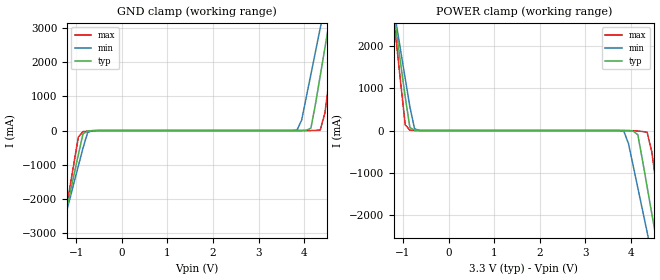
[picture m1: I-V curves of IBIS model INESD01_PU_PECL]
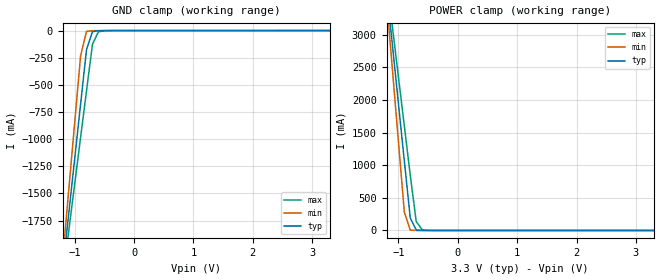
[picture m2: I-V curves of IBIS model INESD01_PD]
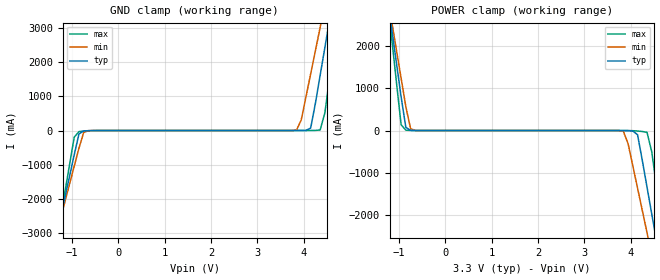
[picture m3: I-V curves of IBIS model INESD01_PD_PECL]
|   This file is an IBIS representation of the   |
|   Integrated Device Technology , Inc.   |
|   ICS87951I   |
|   LOW SKEW, 1-TO-9 DIFFERENTIAL-TO-LVCMOS/LVTTL ZERO DELAY BUFFER   |
[IBIS Ver]   4.1
[File name]   87951i_3v3.ibs
[File Rev]   1.0
[Date]   22 Jun 2009 | Last modified
[Source]   Originated at Integrated Device Technology, Inc.
[Disclaimer]
IDT hereby grants the user of this IBIS model a non-exclusive,
nontransferable license to use this IBIS model under the following terms.
Before using this IBIS model, the user should read this license.
If the user does not accept these terms,  the IBIS model should be
returned to IDT within 30 days.
   The user is granted this license only to use the IBIS model and
is not granted rights to sell, load, rent, lease or license the IBIS
model in whole or in part, or in modified form to anyone other than
user. User may modify the IBIS model to suit its specific
applications but rights to derivative works and such modifications
shall belong to IDT.
   This IBIS model is provided on an "AS IS" basis and IDT makes
absolutely no warranty with respect to the information contained
herein. IDT DISCLAIMS AND CUSTOMER WAIVES ALL WARRANTIES, EXPRESS
OR IMPLIED, INCLUDING WARRANTIES OF MERCHANTABILITY OR FITNESS FOR
A PARTICULAR PURPOSE. The entire risk as to quality and performance
is with the Customer. ACCORDINGLY, IN NO EVENT SHALL THE COMPANY BE
LIABLE FOR ANY DAMAGES, WHETHER IN CONTRACT OR TORT,INCLUDING ANY
LOST PROFITS OR OTHER INCIDENTAL, CONSEQUENTIAL, EXEMPLARY, OR
PUNITIVE DAMAGES ARISING OUT OF THE USE OR APPLICATION OF THE IBIS
model provided in this package. Further, IDT reserves the right to
make changes without notice to any product herein to improve
reliability, function, or design. IDT does not convey any license
under patent rights or any other intellectual property rights,
including those of third parties.
   IDT is not obligated to provide maintenance or support
for the licensed IBIS model.
[Copyright]   Copyright 2003 by Integrated Device Technology , Inc.
[Component]   ICS87951i
[Manufacturer] Integrated Device Technology, Inc.
[Package]
|LQFP32
|lead + wire   typ   min   max
R_pkg   220.4m   212.5m   238m
L_pkg   1.841nH   1.708nH   1.974n
C_pkg   0.316pF   0.2907pF   0.33pF
[Pin] signal_name   model_name   R_pin   L_pin   C_pin
1   VDDA   POWER   238m   1.974n   0.330p
2   EXT_FB   INESD01_PU_PECL   225m   1.841n   0.311p
3   DIV_SELA   INESD01_PD   218m   1.7745n   0.301p
4   DIV_SELB   INESD01_PD   213m   1.708n   0.291p
5   DIV_SELC   INESD01_PD   213m   1.708n   0.291p
6   DIV_SELD   INESD01_PD   218m   1.7745n   0.301p
7   GND   GND   225m   1.841n   0.311p
8   CLK1   INESD01_PU_PECL   238m   1.974n   0.330p
9   nCLK1   INESD01_PD_PECL   238m   1.974n   0.330p
10   MR/nOE   INESD01_PD   225m   1.841n   0.311p
11   VDDO   POWER   218m   1.7745n   0.301p
12   QD4   COUT05   213m   1.708n   0.291p
13   GND   GND   213m   1.708n   0.291p
14   QD3   COUT05   218m   1.7745n   0.301p
15   VDDO   POWER   225m   1.841n   0.311p
16   QD2   COUT05   238m   1.974n   0.330p
17   GND   GND   238m   1.974n   0.330p
18   QD1   COUT05   225m   1.841n   0.311p
19   VDDO   POWER   218m   1.7745n   0.301p
20   QD0   COUT05   213m   1.708n   0.291p
21   GND   GND   213m   1.708n   0.291p
22   QC1   COUT05   218m   1.7745n   0.301p
23   VDDO   POWER   225m   1.841n   0.311p
24   QC0   COUT05   238m   1.974n   0.330p
25   GND   GND   238m   1.974n   0.330p
26   QB   COUT05   225m   1.841n   0.311p
27   VDDO   POWER   218m   1.7745n   0.301p
28   QA   COUT05   213m   1.708n   0.291p
29   GND   GND   213m   1.708n   0.291p
30   CLK0   INESD01_PD_PECL   218m   1.7745n   0.301p
31   PLL_SEL   INESD01_PD   225m   1.841n   0.311p
32   CLK_SEL   INESD01_PD   238m   1.974n   0.330p
[Diff Pin]   inv_pin   vdiff   tdelay_typ   tdelay_min   tdelay_max
8   9   0.30   0   0   0
| Models and submodels in the file (4): INESD01_PU_PECL (Input), INESD01_PD (Input), INESD01_PD_PECL (Input), COUT05 (Output)
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[Model]   INESD01_PU_PECL
Model_type  Input
Polarity   Non-Inverting
Vinl = 0.8V
Vinh = 2.0V
|   typ   min   max
C_comp   2pF   1.5pF   2.5pF
|   typ   min   max
[Voltage range]  3.3V   3.15V   3.45V
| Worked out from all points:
|   GND clamp passes 1 mA (typ) near -0.55 V on its own axis
|   POWER clamp passes 1 mA (typ) near -0.67 V on its own axis
[GND_clamp]
|Voltage   I(typ)   I(min)   I(max)
-3.3V     -15.3A     -13.19A    -18.82A
-1.361V   -3.24A     -3.145A    -3.432A
-1.259V   -2.606A    -2.617A    -2.622A
-952.6mV  -705.4mA   -1.038A    -192.5mA
-850.5mV  -99.96mA   -513.6mA   -31.29mA
-646.4mV  -3.852mA   -3.611mA   -8.361mA
3.844V    64.83uA    13.07mA    7.183uA
4.151V    73.26mA    1.652A     800.8uA
4.355V    1.607A     3.003A     15.37mA
4.559V    3.233A     4.356A     1.553A
4.763V    4.861A     5.711A     3.635A
6.6V      19.56A     17.94A     22.42A
[POWER_clamp]
|Voltage   I(typ)   I(min)   I(max)
-3.3V     19.56A     16.84A     24.11A
-1.259V   3.233A     3.262A     3.235A
-1.157V   2.419A     2.586A     2.194A
-952.6mV  795.8mA    1.236A     137.7mA
-850.5mV  73.26mA    563.1mA    8.081mA
-646.4mV  471.5uA    1.942mA    367.2uA
3.844V    -890.5uA   -18.21mA   -111uA
4.151V    -99.96mA   -1.362A    -11.88mA
4.355V    -1.338A    -2.415A    -41.77mA
4.559V    -2.606A    -3.47A     -1.313A
4.763V    -3.875A    -4.526A    -2.933A
6.6V      -15.3A     -14.05A    -17.51A
[Model]   INESD01_PD
Model_type   Input
Polarity   Non-Inverting
Vinl = 0.80V
Vinh = 2.0V
|   typ   min   max
C_comp   2pF   1.5pF   2.5pF
|   typ   min   max
[Voltage range]  3.3V   3.15V   3.45V
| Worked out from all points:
|   GND clamp passes 1 mA (typ) near -0.55 V on its own axis
|   POWER clamp passes 1 mA (typ) near -0.60 V on its own axis
[GND_clamp]
|Voltage I(typ)   I(min)   I(max)
-3.3V     -12.83A    -15.14A    -11.37A
-1.2V     -2.195A    -2.092A    -2.281A
-1.1V     -1.689A    -1.472A    -1.849A
-900mV    -678.5mA   -232.6mA   -984.8mA
-800mV    -173.9mA   -7.175mA   -553.2mA
-700mV    -9.696mA   -1.052mA   -126mA
-600mV    -1.629mA   -178uA     -11.07mA
-300mV    -10.53uA   -5.678uA   -86.08uA
3.3V      71.13uA    62.11uA    77.58uA
[POWER_clamp]
|Voltage   I(typ)   I(min)   I(max)
-3.3V     22.38A     26.45A     19.82A
-1.2V     3.723A     3.545A     3.874A
-1.1V     2.836A     2.457A     3.116A
-1V       1.949A     1.369A     2.358A
-900mV    1.063A     281.1mA    1.601A
-800mV    191.6mA    5.074mA    844mA
-700mV    8.104mA    204.3uA    138.4mA
-600mV    678.1uA    79.74uA    10.7mA
-400mV    87.44uA    69.65uA    413.2uA
3.3V      -3.041nA   -425fA     -919.9nA
[Model]   INESD01_PD_PECL
Model_type  Input
Polarity   Non-Inverting
Vinl = 0.8V
Vinh = 2.0V
|   typ   min   max
C_comp   2pF   1.5pF   2.5pF
|   typ   min   max
[Voltage range]  3.3V   3.15V   3.45V
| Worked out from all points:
|   GND clamp passes 1 mA (typ) near -0.55 V on its own axis
|   POWER clamp passes 1 mA (typ) near -0.66 V on its own axis
[GND_clamp]
|Voltage   I(typ)   I(min)   I(max)
-2.586V   -10.86A    -9.487A    -13.15A
-1.361V   -3.24A     -3.145A    -3.432A
-1.259V   -2.606A    -2.617A    -2.622A
-952.6mV  -705.3mA   -1.038A    -192.4mA
-850.5mV  -99.9mA    -513.5mA   -31.23mA
-646.4mV  -3.788mA   -3.549mA   -8.297mA
3.844V    129.1uA    13.13mA    71.12uA
4.151V    73.33mA    1.652A     864.7uA
4.355V    1.607A     3.003A     15.44mA
4.559V    3.233A     4.356A     1.553A
4.763V    4.861A     5.711A     3.635A
5.375V    9.757A     9.783A     9.893A
[POWER_clamp]
|Voltage   I(typ)   I(min)   I(max)
-2.177V   10.57A     9.364A     12.62A
-1.157V   2.42A      2.586A     2.194A
-952.6mV  795.8mA    1.237A     137.8mA
-850.5mV  73.33mA    563.2mA    8.145mA
-646.4mV  535.8uA    2.004mA    431.2uA
3.844V    -826.3uA   -18.14mA   -47.07uA
4.151V    -99.9mA    -1.362A    -11.82mA
4.355V    -1.338A    -2.415A    -41.71mA
4.559V    -2.606A    -3.47A     -1.312A
4.661V    -3.24A     -3.998A    -2.123A
4.763V    -3.875A    -4.526A    -2.933A
5.579V    -8.954A    -8.756A    -9.414A
